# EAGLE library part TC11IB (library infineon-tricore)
32-Bit Single-Chip Microcontroller TriCore Family Source: http://www.infineon.com .. TC11IB_DS_v24.pdf
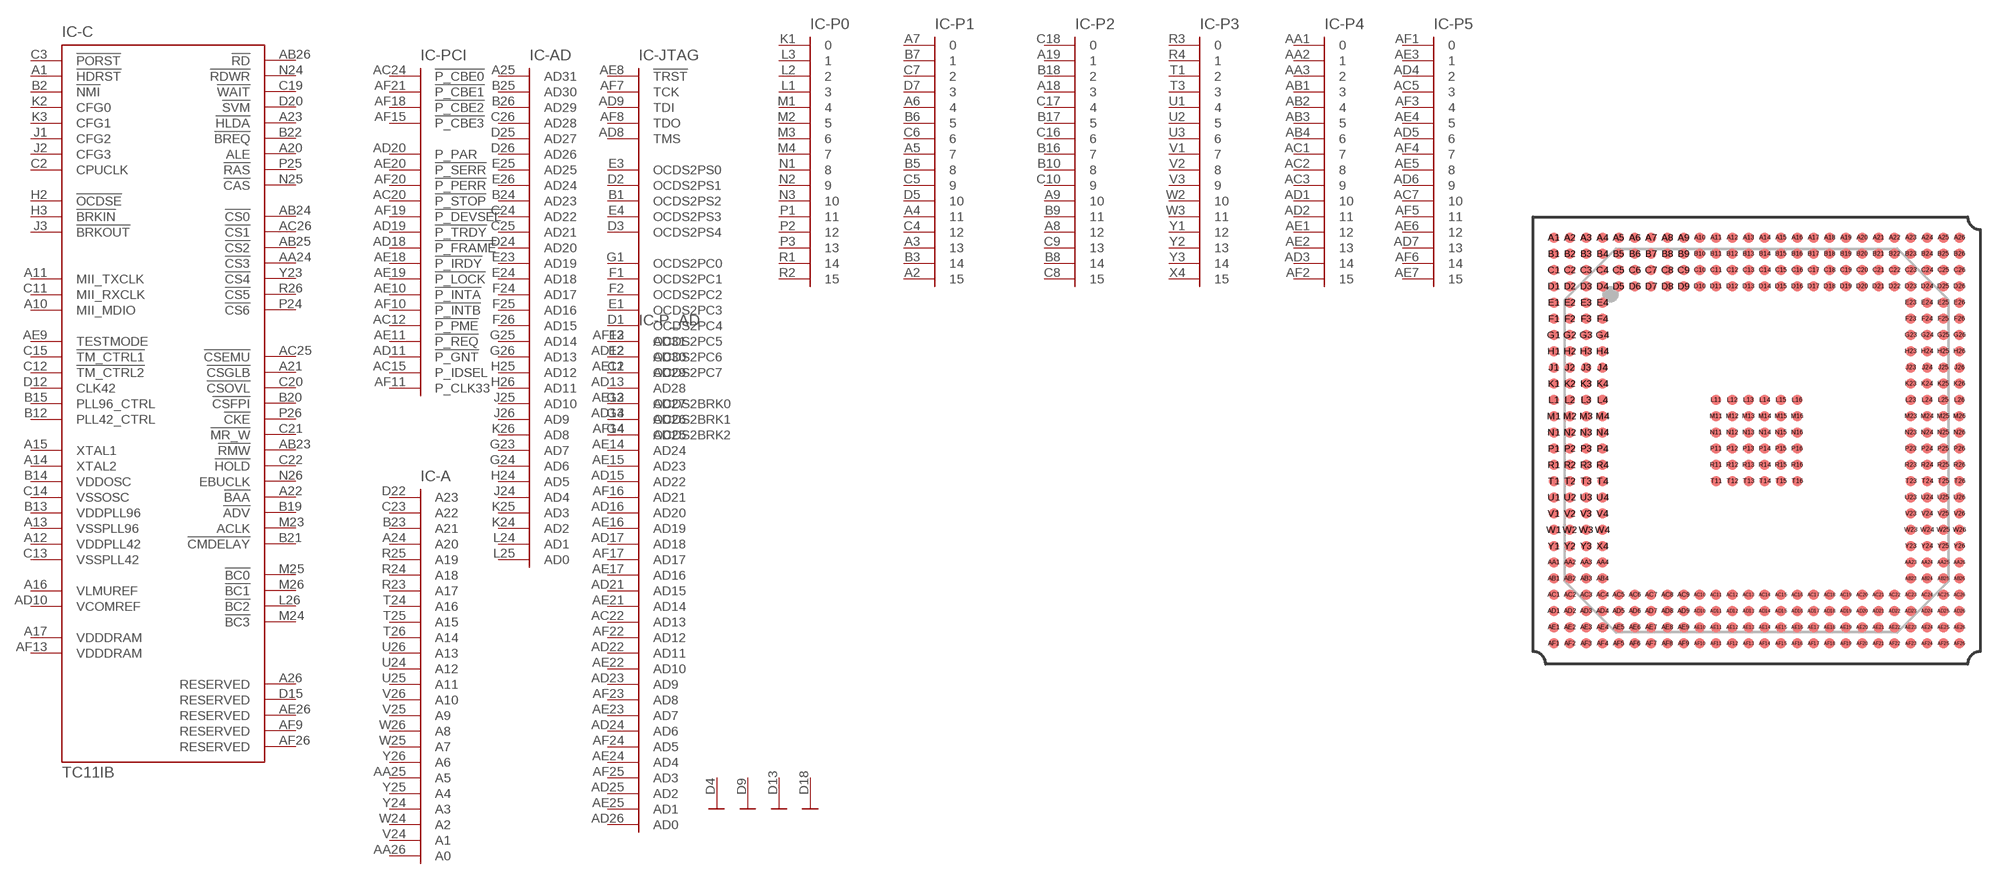
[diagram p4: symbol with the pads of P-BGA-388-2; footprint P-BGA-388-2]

Designator prefix IC; gates -C=TC11IB -PCI=PCI -AD=AD31 -JTAG=ODCS/JTAG -P0=PORT16 -P1=PORT16 -P2=PORT16 -P3=PORT16 -P4=PORT16 -P5=PORT16 -P_AD=AD31 -A=A23 -VSS1=VSS -VSS2=VSS -VSS3=VSS -VSS4=VSS -VSS5=VSS -VSS6=VSS -VSS7=VSS -VSS8=VSS -VSS9=VSS -VSS10=VSS -VSS11=VSS -VSS12=VSS -VSS13=VSS -VSS14=VSS -VSS15=VSS -VSS16=VSS -VSS17=VSS -VSS18=VSS -VSS19=VSS -VSS20=VSS -VSS21=VSS -VSS22=VSS -VSS23=VSS -VSS24=VSS -VSS25=VSS -VSS26=VSS -VSS27=VSS -VSS28=VSS -VSS29=VSS -VSS30=VSS -VSS31=VSS -VSS32=VSS -VSS33=VSS -VSS34=VSS -VSS35=VSS -VSS36=VSS -VSS37=VSS -VSS38=VSS -VSS39=VSS -VSS40=VSS -VSS41=VSS -VSS42=VSS -VSS43=VSS -VSS44=VSS -VSS45=VSS -VSS46=VSS -VSS47=VSS -VSS48=VSS -VSS49=VSS -VSS50=VSS -VSS51=VSS -VSS52=VSS VDDP1=VDDP VDDP2=VDDP VDDP3=VDDP VDDP4=VDDP VDDP5=VDDP VDDP6=VDDP VDDP7=VDDP VDDP8=VDDP VDDP9=VDDP VDDP10=VDDP VDDP11=VDDP VDDP12=VDDP VDDP13=VDDP VDDP14=VDDP VDDP15=VDDP VDDP16=VDDP VDDP17=VDDP VDDP18=VDDP VDDP19=VDDP VDDP20=VDDP VDD1=VDD VDD2=VDD VDD3=VDD VDD4=VDD VDD5=VDD VDD6=VDD VDD7=VDD VDD8=VDD VDD9=VDD VDD10=VDD VDD11=VDD VDD12=VDD VDD13=VDD VDD14=VDD VDD15=VDD VDD16=VDD VDD17=VDD VDD18=VDD VDD19=VDD VDD20=VDD VDD21=VDD

## TC11IB (OC_FARNELL: unknown; OC_NEWARK: unknown)  [P-BGA-388-2]
A1  -C:!HDRST
A2  -P1:15  in
A3  -P1:13  in
A4  -P1:11  in
A5  -P1:7  in
A6  -P1:4  in
A7  -P1:0  in
A8  -P2:12  in
A9  -P2:10  in
A10  -C:MII_MDIO  in
A11  -C:MII_TXCLK  in
A12  -C:VDDPLL42  in
A13  -C:VSSPLL96  in
A14  -C:XTAL2  out
A15  -C:XTAL1  in
A16  -C:VLMUREF  in
A17  -C:VDDDRAM  in
A18  -P2:3  in
A19  -P2:1  in
A20  -C:ALE  out
A21  -C:!CSGLB  out
A22  -C:!BAA  out
A23  -C:!HLDA
A24  -A:A20  out
A25  -AD:AD31
A26  -C:RESERVED  out
AA1  -P4:0  in
AA2  -P4:1  in
AA3  -P4:2  in
AA4  VDD16:VDD  pwr
AA23  VDD17:VDD  pwr
AA24  -C:!CS3  out
AA25  -A:A5  out
AA26  -A:A0  out
AB1  -P4:3  in
AB2  -P4:4  in
AB3  -P4:5  in
AB4  -P4:6  in
AB23  -C:!RMW  out
AB24  -C:!CS0  out
AB25  -C:!CS2  out
AB26  -C:!RD
AC1  -P4:7  in
AC2  -P4:8  in
AC3  -P4:9  in
AC4  -VSS12:VSS  pwr
AC5  -P5:3  in
AC6  VDD18:VDD  pwr
AC7  -P5:10  in
AC8  VDDP16:VDDP  pwr
AC9  -VSS13:VSS  pwr
AC10  VDD19:VDD  pwr
AC11  VDDP17:VDDP  pwr
AC12  -PCI:!P_PME  out
AC13  VDDP18:VDDP  pwr
AC14  -VSS14:VSS  pwr
AC15  -PCI:P_IDSEL  in
AC16  VDDP19:VDDP  pwr
AC17  VDD20:VDD  pwr
AC18  -VSS15:VSS  pwr
AC19  VDDP20:VDDP  pwr
AC20  -PCI:!P_STOP
AC21  VDD21:VDD  pwr
AC22  -P_AD:AD13
AC23  -VSS16:VSS  pwr
AC24  -PCI:!P_CBE0
AC25  -C:!CSEMU  out
AC26  -C:!CS1  out
AD1  -P4:10  in
AD2  -P4:11  in
AD3  -P4:14  in
AD4  -P5:2  in
AD5  -P5:6  in
AD6  -P5:9  in
AD7  -P5:13  in
AD8  -JTAG:TMS  in
AD9  -JTAG:TDI  in
AD10  -C:VCOMREF  in
AD11  -PCI:!P_GNT  in
AD12  -P_AD:AD30
AD13  -P_AD:AD28
AD14  -P_AD:AD26
AD15  -P_AD:AD22
AD16  -P_AD:AD20
AD17  -P_AD:AD18
AD18  -PCI:!P_FRAME
AD19  -PCI:!P_TRDY
AD20  -PCI:P_PAR
AD21  -P_AD:AD15
AD22  -P_AD:AD11
AD23  -P_AD:AD9
AD24  -P_AD:AD6
AD25  -P_AD:AD2
AD26  -P_AD:AD0
AE1  -P4:12  in
AE2  -P4:13  in
AE3  -P5:1  in
AE4  -P5:5  in
AE5  -P5:8  in
AE6  -P5:12  in
AE7  -P5:15  in
AE8  -JTAG:!TRST  in
AE9  -C:TESTMODE  in
AE10  -PCI:!P_INTA  out
AE11  -PCI:!P_REQ  out
AE12  -P_AD:AD29
AE13  -P_AD:AD27
AE14  -P_AD:AD24
AE15  -P_AD:AD23
AE16  -P_AD:AD19
AE17  -P_AD:AD16
AE18  -PCI:!P_IRDY
AE19  -PCI:!P_LOCK
AE20  -PCI:!P_SERR
AE21  -P_AD:AD14
AE22  -P_AD:AD10
AE23  -P_AD:AD7
AE24  -P_AD:AD4
AE25  -P_AD:AD1
AE26  -C:RESERVED
AF1  -P5:0  in
AF2  -P4:15  in
AF3  -P5:4  in
AF4  -P5:7  in
AF5  -P5:11  in
AF6  -P5:14  in
AF7  -JTAG:TCK  in
AF8  -JTAG:TDO  out
AF9  -C:RESERVED
AF10  -PCI:!P_INTB  out
AF11  -PCI:P_CLK33  in
AF12  -P_AD:AD31
AF13  -C:VDDDRAM  in
AF14  -P_AD:AD25
AF15  -PCI:!P_CBE3
AF16  -P_AD:AD21
AF17  -P_AD:AD17
AF18  -PCI:!P_CBE2
AF19  -PCI:!P_DEVSEL
AF20  -PCI:!P_PERR
AF21  -PCI:!P_CBE1
AF22  -P_AD:AD12
AF23  -P_AD:AD8
AF24  -P_AD:AD5
AF25  -P_AD:AD3
AF26  -C:RESERVED
B1  -JTAG:OCDS2PS2  out
B2  -C:!NMI  in
B3  -P1:14  in
B4  VDD4:VDD  pwr
B5  -P1:8  in
B6  -P1:5  in
B7  -P1:1  in
B8  -P2:14  in
B9  -P2:11  in
B10  -P2:8  in
B11  VDD5:VDD  pwr
B12  -C:PLL42_CTRL  out
B13  -C:VDDPLL96  in
B14  -C:VDDOSC  in
B15  -C:PLL96_CTRL  out
B16  -P2:7  in
B17  -P2:5  in
B18  -P2:2  in
B19  -C:!ADV  out
B20  -C:!CSFPI  out
B21  -C:!CMDELAY  in
B22  -C:!BREQ  out
B23  -A:A21  out
B24  -AD:AD23
B25  -AD:AD30
B26  -AD:AD29
C1  -JTAG:OCDS2PC7  out
C2  -C:CPUCLK  out
C3  -C:!PORST  in
C4  -P1:12  in
C5  -P1:9  in
C6  -P1:6  in
C7  -P1:2  in
C8  -P2:15  in
C9  -P2:13  in
C10  -P2:9  in
C11  -C:MII_RXCLK  in
C12  -C:!TM_CTRL2  in
C13  -C:VSSPLL42  in
C14  -C:VSSOSC  in
C15  -C:!TM_CTRL1  in
C16  -P2:6  in
C17  -P2:4  in
C18  -P2:0  in
C19  -C:!WAIT
C20  -C:!CSOVL  out
C21  -C:!MR_W  out
C22  -C:!HOLD  in
C23  -A:A22  out
C24  -AD:AD22
C25  -AD:AD21
C26  -AD:AD28
D1  -JTAG:OCDS2PC4  out
D2  -JTAG:OCDS2PS1  out
D3  -JTAG:OCDS2PS4  out
D4  -VSS1:VSS  pwr
D5  -P1:10  in
D6  VDD6:VDD  pwr
D7  -P1:3  in
D8  VDDP1:VDDP  pwr
D9  -VSS2:VSS  pwr
D10  VDD8:VDD  pwr
D11  VDDP2:VDDP  pwr
D12  -C:CLK42  in
D13  -VSS3:VSS  pwr
D14  VDDP3:VDDP  pwr
D15  -C:RESERVED
D16  VDDP4:VDDP  pwr
D17  VDD9:VDD  pwr
D18  -VSS4:VSS  pwr
D19  VDDP5:VDDP  pwr
D20  -C:!SVM  out
D21  VDD10:VDD  pwr
D22  -A:A23  out
D23  -VSS5:VSS  pwr
D24  -AD:AD20
D25  -AD:AD27
D26  -AD:AD26
E1  -JTAG:OCDS2PC3  out
E2  -JTAG:OCDS2PC6  out
E3  -JTAG:OCDS2PS0  out
E4  -JTAG:OCDS2PS3  out
E23  -AD:AD19
E24  -AD:AD18
E25  -AD:AD25
E26  -AD:AD24
F1  -JTAG:OCDS2PC1  out
F2  -JTAG:OCDS2PC2  out
F3  -JTAG:OCDS2PC5  out
F4  VDD7:VDD  pwr
F23  VDD11:VDD  pwr
F24  -AD:AD17
F25  -AD:AD16
F26  -AD:AD15
G1  -JTAG:OCDS2PC0  out
G2  -JTAG:OCDS2BRK0  out
G3  -JTAG:OCDS2BRK1  out
G4  -JTAG:OCDS2BRK2  out
G23  -AD:AD7
G24  -AD:AD6
G25  -AD:AD14
G26  -AD:AD13
H1  VDD1:VDD  pwr
H2  -C:!OCDSE  in
H3  -C:!BRKIN  in
H4  VDDP6:VDDP  pwr
H23  VDDP7:VDDP  pwr
H24  -AD:AD5
H25  -AD:AD12
H26  -AD:AD11
J1  -C:CFG2
J2  -C:CFG3
J3  -C:!BRKOUT  out
J4  -VSS6:VSS  pwr
J23  -VSS7:VSS  pwr
J24  -AD:AD4
J25  -AD:AD10
J26  -AD:AD9
K1  -P0:0  in
K2  -C:CFG0
K3  -C:CFG1
K4  VDD12:VDD  pwr
K23  VDD13:VDD  pwr
K24  -AD:AD2
K25  -AD:AD3
K26  -AD:AD8
L1  -P0:3  in
L2  -P0:2  in
L3  -P0:1  in
L4  VDDP8:VDDP  pwr
L11  -VSS17:VSS  pwr
L12  -VSS18:VSS  pwr
L13  -VSS19:VSS  pwr
L14  -VSS20:VSS  pwr
L15  -VSS21:VSS  pwr
L16  -VSS22:VSS  pwr
L23  VDDP9:VDDP  pwr
L24  -AD:AD1
L25  -AD:AD0
L26  -C:!BC2
M1  -P0:4  in
M2  -P0:5  in
M3  -P0:6  in
M4  -P0:7  in
M11  -VSS23:VSS  pwr
M12  -VSS24:VSS  pwr
M13  -VSS25:VSS  pwr
M14  -VSS26:VSS  pwr
M15  -VSS27:VSS  pwr
M16  -VSS28:VSS  pwr
M23  -C:ACLK  out
M24  -C:!BC3
M25  -C:!BC0
M26  -C:!BC1
N1  -P0:8  in
N2  -P0:9  in
N3  -P0:10  in
N4  VDDP10:VDDP  pwr
N11  -VSS29:VSS  pwr
N12  -VSS30:VSS  pwr
N13  -VSS31:VSS  pwr
N14  -VSS32:VSS  pwr
N15  -VSS33:VSS  pwr
N16  -VSS34:VSS  pwr
N23  -VSS8:VSS  pwr
N24  -C:!RDWR
N25  -C:!CAS  out
N26  -C:EBUCLK  out
P1  -P0:11  in
P2  -P0:12  in
P3  -P0:13  in
P4  -VSS9:VSS  pwr
P11  -VSS35:VSS  pwr
P12  -VSS36:VSS  pwr
P13  -VSS37:VSS  pwr
P14  -VSS38:VSS  pwr
P15  -VSS39:VSS  pwr
P16  -VSS40:VSS  pwr
P23  VDDP11:VDDP  pwr
P24  -C:!CS6  out
P25  -C:!RAS  out
P26  -C:!CKE  out
R1  -P0:14  in
R2  -P0:15  in
R3  -P3:0  in
R4  -P3:1  in
R11  -VSS41:VSS  pwr
R12  -VSS42:VSS  pwr
R13  -VSS43:VSS  pwr
R14  -VSS44:VSS  pwr
R15  -VSS45:VSS  pwr
R16  -VSS46:VSS  pwr
R23  -A:A17  out
R24  -A:A18  out
R25  -A:A19  out
R26  -C:!CS5  out
T1  -P3:2  in
T2  VDD3:VDD  pwr
T3  -P3:3  in
T4  VDDP12:VDDP  pwr
T11  -VSS47:VSS  pwr
T12  -VSS48:VSS  pwr
T13  -VSS49:VSS  pwr
T14  -VSS50:VSS  pwr
T15  -VSS51:VSS  pwr
T16  -VSS52:VSS  pwr
T23  VDDP13:VDDP  pwr
T24  -A:A16  out
T25  -A:A15  out
T26  -A:A14  out
U1  -P3:4  in
U2  -P3:5  in
U3  -P3:6  in
U4  VDD14:VDD  pwr
U23  VDD15:VDD  pwr
U24  -A:A12  out
U25  -A:A11  out
U26  -A:A13  out
V1  -P3:7  in
V2  -P3:8  in
V3  -P3:9  in
V4  -VSS10:VSS  pwr
V23  -VSS11:VSS  pwr
V24  -A:A1  out
V25  -A:A9  out
V26  -A:A10  out
W1  VDD2:VDD  pwr
W2  -P3:10  in
W3  -P3:11  in
W4  VDDP14:VDDP  pwr
W23  VDDP15:VDDP  pwr
W24  -A:A2  out
W25  -A:A7  out
W26  -A:A8  out
X4  -P3:15  in
Y1  -P3:12  in
Y2  -P3:13  in
Y3  -P3:14  in
Y23  -C:!CS4  out
Y24  -A:A3  out
Y25  -A:A4  out
Y26  -A:A6  out

## Footprint P-BGA-388-2 (pad centres in mm)
P-BGA-388 Plastic Ball Grid Array Package Source: www.infenon.com .. gpa09218.eps.ps
smd 0.8 x 0.8: A1 -15.875,15.875; A2 -14.605,15.875; A3 -13.335,15.875; A4 -12.065,15.875; A5 -10.795,15.875; A6 -9.525,15.875; A7 -8.255,15.875; A8 -6.985,15.875; A9 -5.715,15.875; A10 -4.445,15.875; A11 -3.175,15.875; A12 -1.905,15.875; A13 -0.635,15.875; A14 0.635,15.875; A15 1.905,15.875; A16 3.175,15.875; A17 4.445,15.875; A18 5.715,15.875; A19 6.985,15.875; A20 8.255,15.875; A21 9.525,15.875; A22 10.795,15.875; A23 12.065,15.875; A24 13.335,15.875; A25 14.605,15.875; A26 15.875,15.875; AA1 -15.875,-9.525; AA2 -14.605,-9.525; AA3 -13.335,-9.525; AA4 -12.065,-9.525; AA23 12.065,-9.525; AA24 13.335,-9.525; AA25 14.605,-9.525; AA26 15.875,-9.525; AB1 -15.875,-10.795; AB2 -14.605,-10.795; AB3 -13.335,-10.795; AB4 -12.065,-10.795; AB23 12.065,-10.795; AB24 13.335,-10.795; AB25 14.605,-10.795; AB26 15.875,-10.795; AC1 -15.875,-12.065; AC2 -14.605,-12.065; AC3 -13.335,-12.065; AC4 -12.065,-12.065; AC5 -10.795,-12.065; AC6 -9.525,-12.065; AC7 -8.255,-12.065; AC8 -6.985,-12.065; AC9 -5.715,-12.065; AC10 -4.445,-12.065; AC11 -3.175,-12.065; AC12 -1.905,-12.065; AC13 -0.635,-12.065; AC14 0.635,-12.065; AC15 1.905,-12.065; AC16 3.175,-12.065; AC17 4.445,-12.065; AC18 5.715,-12.065; AC19 6.985,-12.065; AC20 8.255,-12.065; AC21 9.525,-12.065; AC22 10.795,-12.065; AC23 12.065,-12.065; AC24 13.335,-12.065; AC25 14.605,-12.065; AC26 15.875,-12.065; AD1 -15.875,-13.335; AD2 -14.605,-13.335; AD3 -13.335,-13.335; AD4 -12.065,-13.335; AD5 -10.795,-13.335; AD6 -9.525,-13.335; AD7 -8.255,-13.335; AD8 -6.985,-13.335; AD9 -5.715,-13.335; AD10 -4.445,-13.335; AD11 -3.175,-13.335; AD12 -1.905,-13.335; AD13 -0.635,-13.335; AD14 0.635,-13.335; AD15 1.905,-13.335; AD16 3.175,-13.335; AD17 4.445,-13.335; AD18 5.715,-13.335; AD19 6.985,-13.335; AD20 8.255,-13.335; AD21 9.525,-13.335; AD22 10.795,-13.335; AD23 12.065,-13.335; AD24 13.335,-13.335; AD25 14.605,-13.335; AD26 15.875,-13.335; AE1 -15.875,-14.605; AE2 -14.605,-14.605; AE3 -13.335,-14.605; AE4 -12.065,-14.605; AE5 -10.795,-14.605; AE6 -9.525,-14.605; AE7 -8.255,-14.605; AE8 -6.985,-14.605; AE9 -5.715,-14.605; AE10 -4.445,-14.605; AE11 -3.175,-14.605; AE12 -1.905,-14.605; AE13 -0.635,-14.605; AE14 0.635,-14.605; AE15 1.905,-14.605; AE16 3.175,-14.605; AE17 4.445,-14.605; AE18 5.715,-14.605; AE19 6.985,-14.605; AE20 8.255,-14.605; AE21 9.525,-14.605; AE22 10.795,-14.605; AE23 12.065,-14.605; AE24 13.335,-14.605; AE25 14.605,-14.605; AE26 15.875,-14.605; AF1 -15.875,-15.875; AF2 -14.605,-15.875; AF3 -13.335,-15.875; AF4 -12.065,-15.875; AF5 -10.795,-15.875; AF6 -9.525,-15.875; AF7 -8.255,-15.875; AF8 -6.985,-15.875; AF9 -5.715,-15.875; AF10 -4.445,-15.875; AF11 -3.175,-15.875; AF12 -1.905,-15.875; AF13 -0.635,-15.875; AF14 0.635,-15.875; AF15 1.905,-15.875; AF16 3.175,-15.875; AF17 4.445,-15.875; AF18 5.715,-15.875; AF19 6.985,-15.875; AF20 8.255,-15.875; AF21 9.525,-15.875; AF22 10.795,-15.875; AF23 12.065,-15.875; AF24 13.335,-15.875; AF25 14.605,-15.875; AF26 15.875,-15.875; B1 -15.875,14.605; B2 -14.605,14.605; B3 -13.335,14.605; B4 -12.065,14.605; B5 -10.795,14.605; B6 -9.525,14.605; B7 -8.255,14.605; B8 -6.985,14.605; B9 -5.715,14.605; B10 -4.445,14.605; B11 -3.175,14.605; B12 -1.905,14.605; B13 -0.635,14.605; B14 0.635,14.605; B15 1.905,14.605; B16 3.175,14.605; B17 4.445,14.605; B18 5.715,14.605; B19 6.985,14.605; B20 8.255,14.605; B21 9.525,14.605; B22 10.795,14.605; B23 12.065,14.605; B24 13.335,14.605; B25 14.605,14.605; B26 15.875,14.605; C1 -15.875,13.335; C2 -14.605,13.335; C3 -13.335,13.335; C4 -12.065,13.335; C5 -10.795,13.335; C6 -9.525,13.335; C7 -8.255,13.335; C8 -6.985,13.335; C9 -5.715,13.335; C10 -4.445,13.335; C11 -3.175,13.335; C12 -1.905,13.335; C13 -0.635,13.335; C14 0.635,13.335; C15 1.905,13.335; C16 3.175,13.335; C17 4.445,13.335; C18 5.715,13.335; C19 6.985,13.335; C20 8.255,13.335; C21 9.525,13.335; C22 10.795,13.335; C23 12.065,13.335; C24 13.335,13.335; C25 14.605,13.335; C26 15.875,13.335; D1 -15.875,12.065; D2 -14.605,12.065; D3 -13.335,12.065; D4 -12.065,12.065; D5 -10.795,12.065; D6 -9.525,12.065; D7 -8.255,12.065; D8 -6.985,12.065; D9 -5.715,12.065; D10 -4.445,12.065; D11 -3.175,12.065; D12 -1.905,12.065; D13 -0.635,12.065; D14 0.635,12.065; D15 1.905,12.065; D16 3.175,12.065; D17 4.445,12.065; D18 5.715,12.065; D19 6.985,12.065; D20 8.255,12.065; D21 9.525,12.065; D22 10.795,12.065; D23 12.065,12.065; D24 13.335,12.065; D25 14.605,12.065; D26 15.875,12.065; E1 -15.875,10.795; E2 -14.605,10.795; E3 -13.335,10.795; E4 -12.065,10.795; E23 12.065,10.795; E24 13.335,10.795; E25 14.605,10.795; E26 15.875,10.795; F1 -15.875,9.525; F2 -14.605,9.525; F3 -13.335,9.525; F4 -12.065,9.525; F23 12.065,9.525; F24 13.335,9.525; F25 14.605,9.525; F26 15.875,9.525; G1 -15.875,8.255; G2 -14.605,8.255; G3 -13.335,8.255; G4 -12.065,8.255; G23 12.065,8.255; G24 13.335,8.255; G25 14.605,8.255; G26 15.875,8.255; H1 -15.875,6.985; H2 -14.605,6.985; H3 -13.335,6.985; H4 -12.065,6.985; H23 12.065,6.985; H24 13.335,6.985; H25 14.605,6.985; H26 15.875,6.985; J1 -15.875,5.715; J2 -14.605,5.715; J3 -13.335,5.715; J4 -12.065,5.715; J23 12.065,5.715; J24 13.335,5.715; J25 14.605,5.715; J26 15.875,5.715; K1 -15.875,4.445; K2 -14.605,4.445; K3 -13.335,4.445; K4 -12.065,4.445; K23 12.065,4.445; K24 13.335,4.445; K25 14.605,4.445; K26 15.875,4.445; L1 -15.875,3.175; L2 -14.605,3.175; L3 -13.335,3.175; L4 -12.065,3.175; L11 -3.175,3.175; L12 -1.905,3.175; L13 -0.635,3.175; L14 0.635,3.175; L15 1.905,3.175; L16 3.175,3.175; L23 12.065,3.175; L24 13.335,3.175; L25 14.605,3.175; L26 15.875,3.175; M1 -15.875,1.905; M2 -14.605,1.905; M3 -13.335,1.905; M4 -12.065,1.905; M11 -3.175,1.905; M12 -1.905,1.905; M13 -0.635,1.905; M14 0.635,1.905; M15 1.905,1.905; M16 3.175,1.905; M23 12.065,1.905; M24 13.335,1.905; M25 14.605,1.905; M26 15.875,1.905; N1 -15.875,0.635; N2 -14.605,0.635; N3 -13.335,0.635; N4 -12.065,0.635; N11 -3.175,0.635; N12 -1.905,0.635; N13 -0.635,0.635; N14 0.635,0.635; N15 1.905,0.635; N16 3.175,0.635; N23 12.065,0.635; N24 13.335,0.635; N25 14.605,0.635; N26 15.875,0.635; P1 -15.875,-0.635; P2 -14.605,-0.635; P3 -13.335,-0.635; P4 -12.065,-0.635; P11 -3.175,-0.635; P12 -1.905,-0.635; P13 -0.635,-0.635; P14 0.635,-0.635; P15 1.905,-0.635; P16 3.175,-0.635; P23 12.065,-0.635; P24 13.335,-0.635; P25 14.605,-0.635; P26 15.875,-0.635; R1 -15.875,-1.905; R2 -14.605,-1.905; R3 -13.335,-1.905; R4 -12.065,-1.905; R11 -3.175,-1.905; R12 -1.905,-1.905; R13 -0.635,-1.905; R14 0.635,-1.905; R15 1.905,-1.905; R16 3.175,-1.905; R23 12.065,-1.905; R24 13.335,-1.905; R25 14.605,-1.905; R26 15.875,-1.905; T1 -15.875,-3.175; T2 -14.605,-3.175; T3 -13.335,-3.175; T4 -12.065,-3.175; T11 -3.175,-3.175; T12 -1.905,-3.175; T13 -0.635,-3.175; T14 0.635,-3.175; T15 1.905,-3.175; T16 3.175,-3.175; T23 12.065,-3.175; T24 13.335,-3.175; T25 14.605,-3.175; T26 15.875,-3.175; U1 -15.875,-4.445; U2 -14.605,-4.445; U3 -13.335,-4.445; U4 -12.065,-4.445; U23 12.065,-4.445; U24 13.335,-4.445; U25 14.605,-4.445; U26 15.875,-4.445; V1 -15.875,-5.715; V2 -14.605,-5.715; V3 -13.335,-5.715; V4 -12.065,-5.715; V23 12.065,-5.715; V24 13.335,-5.715; V25 14.605,-5.715; V26 15.875,-5.715; W1 -15.875,-6.985; W2 -14.605,-6.985; W3 -13.335,-6.985; W4 -12.065,-6.985; W23 12.065,-6.985; W24 13.335,-6.985; W25 14.605,-6.985; W26 15.875,-6.985; X4 -12.065,-8.255; Y1 -15.875,-8.255; Y2 -14.605,-8.255; Y3 -13.335,-8.255; Y23 12.065,-8.255; Y24 13.335,-8.255; Y25 14.605,-8.255; Y26 15.875,-8.255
